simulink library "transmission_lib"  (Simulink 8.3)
settings: Solver=ode45  StartTime=0.0  StopTime=10.0  RelTol=1e-3
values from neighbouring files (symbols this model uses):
  dual_clutch = class_REVS_dual_clutch    [class_REVS_DCT_transmission.m]
  electric = class_REVS_electric(engine)    [electric_standard_car.m]
  gear = class_REVS_gearbox    [class_REVS_AMT_transmission.m]    (also in class_REVS_AT_transmission.m; class_REVS_CVT_transmission.m)
  torque_converter = class_REVS_torque_converter    [class_REVS_AT_transmission.m]    (also in class_REVS_CVT_transmission.m)
  transmission = class_REVS_AT_transmission    [transmission_6AT.m]    (also in transmission_8DCT.m = class_REVS_DCT_transmission; transmission_CVT.m = class_REVS_CVT_transmission)
undefined symbols (not defined in the file or in its folder): clutch, convert, gear_strategy, InitialSpeed_radps, LoadSource, SpeedSource, Value
libraries: general_lib x129, simulink x57, transmission_lib x50, audit_lib x11
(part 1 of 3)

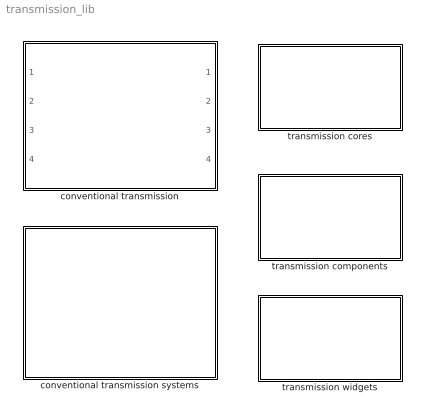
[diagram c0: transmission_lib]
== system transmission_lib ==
  conventional transmission : Subsystem  Variant=on
  conventional transmission systems : Subsystem
  transmission components : Subsystem
  transmission cores : Subsystem
  transmission widgets : Subsystem

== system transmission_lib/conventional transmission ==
  note: 1) Only subsystems can be added as variant choices at this level 2) Blocks cannot be connected at this level as connectivity is automatically determined at simulation, based on the active variant
  system_bus : Inport
  trq_in_Nm : Inport  Port=2
  iner_in_kgm2 : Inport  Port=3
  spd_out_radps : Inport  Port=4
  CVT transmission. system : transmission_lib/conventional transmission systems/CVT transmission system  VariantControl=transmission_type == enum_transmission_type.CVT
  automatic transmission system : transmission_lib/conventional transmission systems/automatic transmission system  VariantControl=transmission_type == enum_transmission_type.automatic
  dct transmission system : transmission_lib/conventional transmission systems/dct transmission system  VariantControl=transmission_type == enum_transmission_type.DCT
  bus_out : Outport
  trq_out_Nm : Outport  Port=2
  iner_out_kgm2 : Outport  Port=3
  spd_in_radps : Outport  Port=4

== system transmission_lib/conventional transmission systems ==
  CVT trans control : Subsystem  VariantControl=variants_trans_control_default
  CVT transmission system : Subsystem  VariantControl=transmission_type == enum_transmission_type.CVT
  automatic trans control : Subsystem  VariantControl=variants_trans_control_default
  automatic transmission system : Subsystem  VariantControl=transmission_type == enum_transmission_type.automatic
  dct trans control : Subsystem  VariantControl=variants_trans_control_manual
  dct transmission system : Subsystem  VariantControl=transmission_type == enum_transmission_type.DCT

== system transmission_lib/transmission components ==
  clutch : Subsystem
  dual clutch module : Subsystem
  gearbox : Subsystem
  simple gear : Subsystem
  torque converter : Subsystem

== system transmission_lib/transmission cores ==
  automatic core control : Subsystem  VariantControl=variants_trans_automatic
  automatic transmission core : Subsystem  VariantControl=variants_trans_automatic
  core control : Subsystem  Variant=on
  dct core control : Subsystem  VariantControl=variants_trans_dct
  dct transmission core : Subsystem  VariantControl=variants_trans_manual
  transmission cores : Subsystem  Variant=on

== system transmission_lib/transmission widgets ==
  auto neutral logic : Subsystem
  delayed lockup : Subsystem
  engage target speed calc : Subsystem
  gear select : Subsystem  Variant=on
  gear select variants : Subsystem
  load select : Subsystem
  lockup select : Subsystem  Variant=on
  lockup select variants : Subsystem
  low speed clutch engagement : Subsystem
  shift counter : Subsystem
  speed select : Subsystem
  thermal model : Subsystem  Variant=on
  thermal variants : Subsystem

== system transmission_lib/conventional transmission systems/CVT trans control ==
  system_bus : Inport
  Auto Neutral : Product  Inputs=**
  Bus Creator : BusCreator  Inputs=10
  Bus Selector : BusSelector  OutputSignals=driver.driver_acl_norm
  Bus Selector1 : BusSelector  OutputSignals=powertrain.trans.core.gearbox.gb_curr_gear
  Compare To Zero : simulink/Logic and Bit Operations/Compare To Zero  relop=>  OutDataTypeStr=boolean  ZeroCross=off
  Logical Operator1 : Logic  Operator=NOT  AllPortsSameDT=off  OutDataTypeStr=boolean
  auto neutral logic : transmission_lib/transmission widgets/auto neutral logic
  comp_iner_enable1 : Constant  Value=Inf
  driver acl to eng des acl : Gain
  gb curr gear to tans curr gear : Gain
  gear select : transmission_lib/transmission widgets/gear select
  line pressure control : Subsystem
  lockup select : transmission_lib/transmission widgets/lockup select
  to datalog : general_lib/to datalog  VarName=transmission__torque_converter_clutch_command_norm  WorkspaceName=datalog__transmission__torque_converter_clutch_command_norm  VerboseLevel=1  VerboseSignal=REVS.verbose
  to datalog1 : general_lib/to datalog  VarName=transmission__selected_gear_num  WorkspaceName=datalog__transmission__selected_gear_num  VerboseLevel=0  VerboseSignal=REVS.verbose
  to datalog2 : general_lib/to datalog  VarName=transmission__command_line_pressure_bar  WorkspaceName=datalog__transmission__command_line_pressure_bar  VerboseLevel=1  VerboseSignal=REVS.verbose
  to datalog5 : general_lib/to datalog  VarName=transmission__current_gear  WorkspaceName=datalog__transmission__current_gear  VerboseLevel=1  VerboseSignal=REVS.verbose
  trans des eng spd : Constant  Value=0
  trans des eng spd1 : Constant  Value=0
  upshift inertia compensation : Subsystem
  bus_out : Outport
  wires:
  auto neutral logic/1 -> Logical Operator1/1
  gear select/1 -> Auto Neutral/1
  Logical Operator1/1 -> Auto Neutral/2
  gb curr gear to tans curr gear/1 -> Bus Creator/9, to datalog5/1  "trans_curr_gear"
  line pressure control/1(cmd_line_press_bar) -> Bus Creator/8, to datalog2/1  "gb_line_press_bar"
  comp_iner_enable1/1 -> Bus Creator/7  "eng_des_load_limit_Nm"
  upshift inertia compensation/1(comp_iner_enable) -> Bus Creator/6  "eng_comp_iner_enable"
  Bus Selector1/1 -> lockup select/1, gb curr gear to tans curr gear/1  "<gb_curr_gear>"
  Bus Selector/1 -> driver acl to eng des acl/1  "<driver_acl_norm>"
  Auto Neutral/1 -> to datalog1/1, Compare To Zero/1, Bus Creator/1  "gear_num"
  system_bus/1 -> Bus Selector1/1, line pressure control/1(system_bus), upshift inertia compensation/1(system_bus), Bus Selector/1, lockup select/2, auto neutral logic/1, gear select/1
  Bus Creator/1 -> bus_out/1  "ctrl"
  lockup select/1 -> Bus Creator/3, to datalog/1  "tcc_lockup_cmd_bool"
  driver acl to eng des acl/1 -> Bus Creator/5  "eng_des_acl_norm"
  trans des eng spd/1 -> Bus Creator/4  "eng_des_spd_radps"
  Compare To Zero/1 -> Bus Creator/2  "driveline_engaged_bool"
  trans des eng spd1/1 -> Bus Creator/10  "trans_shift_in_prog"

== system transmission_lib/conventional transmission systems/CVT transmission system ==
  system_bus : Inport
  trq_in_Nm : Inport  Port=2
  iner_in_kgm2 : Inport  Port=3
  spd_out_radps : Inport  Port=4
  Bus Creator : BusCreator
  CVT trans control : transmission_lib/conventional transmission systems/CVT trans control  VariantControl=variants_trans_control_default
  automatic transmission core : transmission_lib/transmission cores/automatic transmission core  VariantControl=variants_trans_automatic
  result work : general_lib/result work  ResultSignalName=transmission_output_pos_work_kJ
  thermal model : transmission_lib/transmission widgets/thermal model
  to datalog : general_lib/to datalog  VarName=transmission.output_torque_Nm  WorkspaceName=datalog__transmission__output_torque_Nm  VerboseLevel=0  VerboseSignal=REVS.verbose
  to datalog1 : general_lib/to datalog  VarName=transmission.output_inertia_kgm2  WorkspaceName=datalog__transmission__output_inertia_kgm2  VerboseLevel=0  VerboseSignal=REVS.verbose
  to datalog2 : general_lib/to datalog  VarName=transmission.output_speed_radps  WorkspaceName=datalog__transmission__output_speed_radps  VerboseLevel=0  VerboseSignal=REVS.verbose
  torque converter : transmission_lib/transmission components/torque converter  base_name=torque_converter  torque_converter=transmission.torque_converter  pump_loss_Nm=transmission.pump_loss_Nm  pump_loss_base_name=torque_converter__pumploss  InitialSpeed_radps=0
  bus_out : Outport
  trq_out_Nm : Outport  Port=2
  iner_out_kgm2 : Outport  Port=3
  spd_in_radps : Outport  Port=4
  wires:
  spd_out_radps/1 -> to datalog2/1, automatic transmission core/4, result work/2
  torque converter/1 -> Bus Creator/3  "trq_conv"
  Bus Creator/1 -> torque converter/1, automatic transmission core/1, bus_out/1  "trans"
  system_bus/1 -> thermal model/1, CVT trans control/1
  CVT trans control/1 -> Bus Creator/1  "ctrl"
  automatic transmission core/1 -> Bus Creator/4  "core"
  automatic transmission core/2 -> to datalog/1, trq_out_Nm/1, result work/1
  automatic transmission core/3 -> result work/3, to datalog1/1, iner_out_kgm2/1
  trq_in_Nm/1 -> torque converter/2
  iner_in_kgm2/1 -> torque converter/3
  torque converter/2 -> automatic transmission core/2
  torque converter/3 -> automatic transmission core/3
  torque converter/4 -> spd_in_radps/1
  automatic transmission core/4 -> torque converter/4
  thermal model/1 -> Bus Creator/2  "therm"

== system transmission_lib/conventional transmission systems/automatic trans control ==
  system_bus : Inport
  Bus Creator : BusCreator  Inputs=10
  Bus Selector1 : BusSelector  OutputSignals=powertrain.trans.core.gearbox.gb_curr_gear
  Bus Selector2 : BusSelector  OutputSignals=driver.driver_acl_norm
  Compare To Zero : simulink/Logic and Bit Operations/Compare To Zero  relop=>  OutDataTypeStr=boolean  ZeroCross=off
  Divide : Product  Inputs=**
  Logical Operator1 : Logic  Operator=NOT  AllPortsSameDT=off  OutDataTypeStr=boolean
  Saturation : Saturate  UpperLimit=1  LowerLimit=-1
  Sum : Sum  Inputs=+-
  auto neutral logic : transmission_lib/transmission widgets/auto neutral logic
  comp_iner_enable1 : Constant  Value=Inf
  driver acl to eng des acl : Gain
  gb curr gear to tans curr gear : Gain
  gear select : transmission_lib/transmission widgets/gear select
  line pressure control : Subsystem
  lockup select : transmission_lib/transmission widgets/lockup select
  shift counter : transmission_lib/transmission widgets/shift counter
  to datalog : general_lib/to datalog  VarName=transmission__torque_converter_clutch_command_norm  WorkspaceName=datalog__transmission__torque_converter_clutch_command_norm  VerboseLevel=1  VerboseSignal=REVS.verbose
  to datalog1 : general_lib/to datalog  VarName=transmission__selected_gear_num  WorkspaceName=datalog__transmission__selected_gear_num  VerboseLevel=0  VerboseSignal=REVS.verbose
  to datalog2 : general_lib/to datalog  VarName=transmission__command_line_pressure_bar  WorkspaceName=datalog__transmission__command_line_pressure_bar  VerboseLevel=1  VerboseSignal=REVS.verbose
  to datalog5 : general_lib/to datalog  VarName=transmission__current_gear  WorkspaceName=datalog__transmission__current_gear  VerboseLevel=1  VerboseSignal=REVS.verbose
  trans des eng spd : Constant  Value=0
  upshift inertia compensation : Subsystem
  bus_out : Outport
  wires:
  Saturation/1 -> Bus Creator/9  "trans_shift_in_prog"
  Sum/1 -> Saturation/1
  Logical Operator1/1 -> Divide/2
  auto neutral logic/1 -> Logical Operator1/1
  gear select/1 -> Divide/1, to datalog1/1
  Compare To Zero/1 -> Bus Creator/2  "driveline_engaged_bool"
  trans des eng spd/1 -> Bus Creator/6  "eng_des_spd_radps"
  driver acl to eng des acl/1 -> Bus Creator/5  "eng_des_acl_norm"
  lockup select/1 -> to datalog/1, Bus Creator/3  "tcc_lockup_cmd_bool"
  Bus Creator/1 -> bus_out/1  "ctrl"
  system_bus/1 -> Bus Selector2/1, line pressure control/1(system_bus), Bus Selector1/1, upshift inertia compensation/1(system_bus), lockup select/2, auto neutral logic/1, gear select/1
  Divide/1 -> shift counter/1, Sum/1, Compare To Zero/1, Bus Creator/1  "gear_num"
  comp_iner_enable1/1 -> Bus Creator/7  "eng_des_load_limit_Nm"
  line pressure control/1(cmd_line_press_bar) -> Bus Creator/8, to datalog2/1  "gb_line_press_bar"
  gb curr gear to tans curr gear/1 -> Sum/2, Bus Creator/10, to datalog5/1  "trans_curr_gear"
  Bus Selector1/1 -> gb curr gear to tans curr gear/1, lockup select/1  "<gb_curr_gear>"
  Bus Selector2/1 -> driver acl to eng des acl/1  "<driver_acl_norm>"
  upshift inertia compensation/1(comp_iner_enable) -> Bus Creator/4  "eng_comp_iner_enable"

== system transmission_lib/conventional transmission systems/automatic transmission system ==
  system_bus : Inport
  trq_in_Nm : Inport  Port=2
  iner_in_kgm2 : Inport  Port=3
  spd_out_radps : Inport  Port=4
  Bus Creator : BusCreator
  automatic trans control : transmission_lib/conventional transmission systems/automatic trans control  VariantControl=variants_trans_control_default
  automatic transmission core : transmission_lib/transmission cores/automatic transmission core  VariantControl=variants_trans_automatic
  result work : general_lib/result work  ResultSignalName=transmission_output_pos_work_kJ
  thermal model : transmission_lib/transmission widgets/thermal model
  to datalog : general_lib/to datalog  VarName=transmission.output_torque_Nm  WorkspaceName=datalog__transmission__output_torque_Nm  VerboseLevel=0  VerboseSignal=REVS.verbose
  to datalog1 : general_lib/to datalog  VarName=transmission.output_inertia_kgm2  WorkspaceName=datalog__transmission__output_inertia_kgm2  VerboseLevel=0  VerboseSignal=REVS.verbose
  to datalog2 : general_lib/to datalog  VarName=transmission.output_speed_radps  WorkspaceName=datalog__transmission__output_speed_radps  VerboseLevel=0  VerboseSignal=REVS.verbose
  torque converter : transmission_lib/transmission components/torque converter  base_name=torque_converter  torque_converter=transmission.torque_converter  pump_loss_Nm=transmission.pump_loss_Nm  pump_loss_base_name=torque_converter__pumploss  InitialSpeed_radps=0
  bus_out : Outport
  trq_out_Nm : Outport  Port=2
  iner_out_kgm2 : Outport  Port=3
  spd_in_radps : Outport  Port=4
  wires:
  torque converter/1 -> Bus Creator/3  "trq_conv"
  Bus Creator/1 -> automatic transmission core/1, torque converter/1, bus_out/1  "trans"
  system_bus/1 -> thermal model/1, automatic trans control/1
  automatic trans control/1 -> Bus Creator/1  "ctrl"
  automatic transmission core/1 -> Bus Creator/4  "core"
  automatic transmission core/2 -> trq_out_Nm/1, result work/1, to datalog/1
  automatic transmission core/3 -> to datalog1/1, result work/3, iner_out_kgm2/1
  trq_in_Nm/1 -> torque converter/2
  iner_in_kgm2/1 -> torque converter/3
  torque converter/2 -> automatic transmission core/2
  torque converter/3 -> automatic transmission core/3
  spd_out_radps/1 -> automatic transmission core/4, result work/2, to datalog2/1  "trans_spd_out_radps"
  torque converter/4 -> spd_in_radps/1
  automatic transmission core/4 -> torque converter/4
  thermal model/1 -> Bus Creator/2  "therm"

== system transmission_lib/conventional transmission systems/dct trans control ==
  system_bus : Inport
  Bus Creator : BusCreator  Inputs=7
  Bus Selector : BusSelector  OutputSignals=powertrain.engine.eng_spd_radps,powertrain.trans.core.trans_spd_out_radps,driver.driver_acl_norm,driver.driver_brk_norm,powertrain.trans.ctrl.core_ctl.trans_shift_in_prog,powertrain.trans.core.dual_clutch.dct_capacity_Nm
  Bus Selector1 : BusSelector  OutputSignals=trans_curr_gear
  Compare To Zero : simulink/Logic and Bit Operations/Compare To Zero  relop=~=  OutDataTypeStr=boolean  ZeroCross=off
  Product2 : Product
  Saturation : Saturate  UpperLimit=1  LowerLimit=0
  dct cap to load limit : Gain
  dct core control : transmission_lib/transmission cores/dct core control  VariantControl=variants_trans_dct
  driver acl to eng des acl : Gain
  gear ratio : LookupNDDirect  NumberOfTableDimensions=1  Table=transmission.gear.ratio
  gear select : transmission_lib/transmission widgets/gear select
  low speed clutch engagement1 : transmission_lib/transmission widgets/low speed clutch engagement  clutch=transmission.control
  shift counter : transmission_lib/transmission widgets/shift counter
  trans des eng spd : Constant  Value=0
  bus_out : Outport
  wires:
  Bus Selector/6 -> dct cap to load limit/1  "<dct_capacity_Nm>"
  Bus Selector/5 -> Saturation/1  "<trans_shift_in_prog>"
  dct cap to load limit/1 -> Bus Creator/7  "eng_des_load_limit_Nm"
  gear ratio/1 -> Product2/1
  Bus Selector/2 -> Product2/2  "<trans_spd_out_radps>"
  Bus Selector/3 -> low speed clutch engagement1/3, driver acl to eng des acl/1  "<driver_acl_norm>"
  system_bus/1 -> Bus Selector/1, dct core control/1, gear select/1
  Bus Creator/1 -> bus_out/1  "ctrl"
  trans des eng spd/1 -> Bus Creator/5  "eng_des_spd_radps"
  driver acl to eng des acl/1 -> Bus Creator/4  "eng_des_acl_norm"
  Bus Selector/1 -> low speed clutch engagement1/1  "<eng_spd_radps>"
  Product2/1 -> low speed clutch engagement1/2
  Bus Selector/4 -> low speed clutch engagement1/4  "<driver_brk_norm>"
  Saturation/1 -> Bus Creator/6  "eng_comp_iner_enable"
  Compare To Zero/1 -> low speed clutch engagement1/6
  dct core control/1 -> Bus Selector1/1, Bus Creator/3  "core_ctl"
  low speed clutch engagement1/1 -> Bus Creator/1  "clutch_cmd_norm"
  gear select/1 -> gear ratio/1, Bus Creator/2, Compare To Zero/1, low speed clutch engagement1/5  "gear_num"
  Bus Selector1/1 -> shift counter/1  "<trans_curr_gear>"

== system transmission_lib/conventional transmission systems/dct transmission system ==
  system_bus : Inport
  trq_in_Nm : Inport  Port=2
  iner_in_kgm2 : Inport  Port=3
  spd_out_radps : Inport  Port=4
  Bus Creator : BusCreator  Inputs=3
  dct trans control : transmission_lib/conventional transmission systems/dct trans control  VariantControl=variants_trans_control_manual
  dct transmission core : transmission_lib/transmission cores/dct transmission core  VariantControl=variants_trans_manual
  result work : general_lib/result work  ResultSignalName=transmission_output_pos_work_kJ
  thermal model : transmission_lib/transmission widgets/thermal model
  to datalog : general_lib/to datalog  VarName=transmission.output_torque_Nm  WorkspaceName=datalog__transmission__output_torque_Nm  VerboseLevel=0  VerboseSignal=REVS.verbose
  to datalog1 : general_lib/to datalog  VarName=transmission.output_inertia_kgm2  WorkspaceName=datalog__transmission__output_inertia_kgm2  VerboseLevel=0  VerboseSignal=REVS.verbose
  to datalog2 : general_lib/to datalog  VarName=transmission.output_speed_radps  WorkspaceName=datalog__transmission__output_speed_radps  VerboseLevel=0  VerboseSignal=REVS.verbose
  bus_out : Outport
  trq_out_Nm : Outport  Port=2
  iner_out_kgm2 : Outport  Port=3
  spd_in_radps : Outport  Port=4
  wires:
  iner_in_kgm2/1 -> dct transmission core/3
  spd_out_radps/1 -> to datalog2/1, result work/2, dct transmission core/4
  trq_in_Nm/1 -> dct transmission core/2
  dct transmission core/4 -> spd_in_radps/1
  dct transmission core/3 -> result work/3, to datalog1/1, iner_out_kgm2/1
  dct transmission core/2 -> trq_out_Nm/1, result work/1, to datalog/1
  system_bus/1 -> dct trans control/1, thermal model/1
  dct trans control/1 -> Bus Creator/1  "ctrl"
  dct transmission core/1 -> Bus Creator/3  "core"
  thermal model/1 -> Bus Creator/2  "therm"
  Bus Creator/1 -> dct transmission core/1, bus_out/1  "trans"

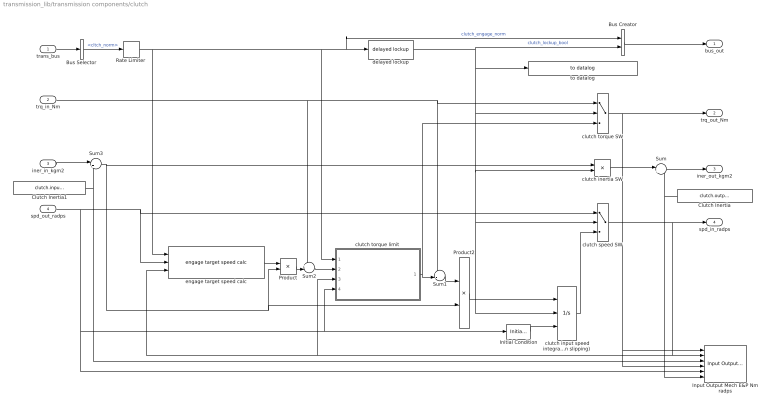
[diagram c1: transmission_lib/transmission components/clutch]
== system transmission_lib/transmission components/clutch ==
  trans_bus : Inport
  trq_in_Nm : Inport  Port=2
  iner_in_kgm2 : Inport  Port=3
  spd_out_radps : Inport  Port=4
  " clutch input speed integrator  (integrate when slipping)" : Integrator  ExternalReset=falling  InitialConditionSource=external  LimitOutput=on  UpperSaturationLimit=Inf  LowerSaturationLimit=0
  Bus Creator : BusCreator  Inputs=2
  Bus Selector : BusSelector  OutputSignals=cltch_norm
  Clutch Inertia : Constant  Value=clutch.output_inertia_kgm2
  Clutch Inertia1 : Constant  Value=clutch.input_inertia_kgm2
  Initial Condition : general_lib/Initial Condition  InitialValue=InitialSpeed_radps
  Input Output Mech E&P Nm radps : audit_lib/Input Output Mech E&P Nm radps  base_name=clutch  VerboseSignal=REVS.verbose
  Product : Product
  Product2 : Product  Inputs=*/
  Rate Limiter : RateLimiter  RisingSlewLimit=1/clutch.engage_duration_secs  FallingSlewLimit=-inf  SampleTimeMode=inherited
  Sum : Sum  Inputs=|++
  Sum1 : Sum  Inputs=+-|
  Sum2 : Sum  Inputs=+-|
  Sum3 : Sum  Inputs=|++
  clutch inertia SW : Product
  clutch speed SW : Switch  Threshold=1
  clutch torque SW : Switch  Threshold=1
  clutch torque limit : Subsystem
  delayed lockup : transmission_lib/transmission widgets/delayed lockup
  engage target speed calc : transmission_lib/transmission widgets/engage target speed calc
  to datalog : general_lib/to datalog  VarName=transmission__clutch_lockup_bool  WorkspaceName=datalog__transmission__clutch_lockup_bool  VerboseLevel=1  VerboseSignal=REVS.verbose
  bus_out : Outport
  trq_out_Nm : Outport  Port=2
  iner_out_kgm2 : Outport  Port=3
  spd_in_radps : Outport  Port=4
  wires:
  Rate Limiter/1 -> clutch torque limit/1(engage), Bus Creator/1, delayed lockup/1, engage target speed calc/1  "clutch_engage_norm"
  delayed lockup/1 -> clutch inertia SW/2, " clutch input speed integrator  (integrate when slipping)"/2, clutch speed SW/2, clutch torque SW/2, to datalog/1, Bus Creator/2  "clutch_lockup_bool"
  Product2/1 -> " clutch input speed integrator  (integrate when slipping)"/1
  Product/1 -> Sum2/2
  spd_out_radps/1 -> clutch speed SW/1, engage target speed calc/2, Initial Condition/1, clutch torque limit/4(output_speed_radps), Input Output Mech E&P Nm radps/5
  " clutch input speed integrator  (integrate when slipping)"/1 -> clutch speed SW/3
  trq_in_Nm/1 -> Sum1/1, clutch torque SW/1, Sum2/1
  Sum3/1 -> clutch inertia SW/1, Product/2, Product2/2
  engage target speed calc/1 -> Product/1
  Sum1/1 -> Product2/1
  clutch speed SW/1 -> clutch torque limit/3(input_speed_radps), engage target speed calc/3, Input Output Mech E&P Nm radps/2, spd_in_radps/1
  clutch torque SW/1 -> trq_out_Nm/1, Input Output Mech E&P Nm radps/4, Input Output Mech E&P Nm radps/1
  trans_bus/1 -> Bus Selector/1
  clutch inertia SW/1 -> Sum/1
  Sum/1 -> iner_out_kgm2/1
  Clutch Inertia/1 -> Input Output Mech E&P Nm radps/6, Sum/2
  iner_in_kgm2/1 -> Sum3/1
  Clutch Inertia1/1 -> Input Output Mech E&P Nm radps/3, Sum3/2
  Initial Condition/1 -> " clutch input speed integrator  (integrate when slipping)"/3
  clutch torque limit/1(lim_transmit_torque_Nm) -> Sum1/2, clutch torque SW/3
  Sum2/1 -> clutch torque limit/2("req_transmit_torque_Nm ")
  Bus Creator/1 -> bus_out/1
  Bus Selector/1 -> Rate Limiter/1  "<cltch_norm>"

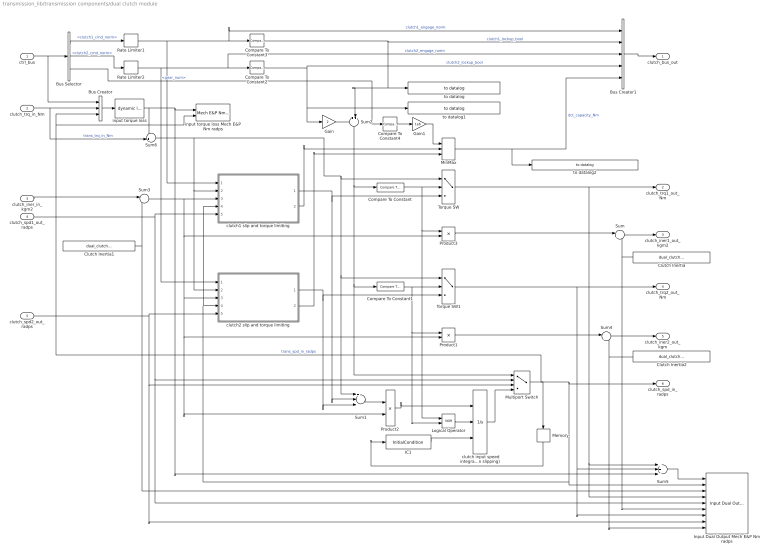
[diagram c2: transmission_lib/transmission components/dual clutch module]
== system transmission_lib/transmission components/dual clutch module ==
  ctrl_bus : Inport
  clutch_trq_in_Nm : Inport  Port=2
  clutch_iner_in_kgm2 : Inport  Port=3
  clutch_spd1_out_radps : Inport  Port=4
  clutch_spd2_out_radps : Inport  Port=5
  " clutch input speed integrator  (integrate when slipping)" : Integrator  ExternalReset=rising  InitialConditionSource=external  LimitOutput=on  UpperSaturationLimit=Inf  LowerSaturationLimit=0
  Bus Creator : BusCreator  Inputs=3
  Bus Creator1 : BusCreator  Inputs=5
  Bus Selector : BusSelector  OutputSignals=ctrl.core_ctl.clutch1_cmd_norm,ctrl.core_ctl.clutch2_cmd_norm,ctrl.gear_num
  Clutch Inertia : Constant  Value=dual_clutch.output1_inertia_kgm2
  Clutch Inertia1 : Constant  Value=dual_clutch.input_inertia_kgm2
  Clutch Inertia2 : Constant  Value=dual_clutch.output2_inertia_kgm2
  Compare To Constant{,2..4} (4 alike) : simulink/Logic and Bit Operations/Compare To Constant  relop===  const=1  OutDataTypeStr=boolean
  Compare To Constant1 : simulink/Logic and Bit Operations/Compare To Constant  relop===  const=2  OutDataTypeStr=boolean
  Gain : Gain  Gain=2
  Gain1 : Gain  Gain=1e6
  IC1 : InitialCondition  Value=InitialSpeed_radps
  Input Dual Output Mech E&P Nm radps : audit_lib/Input Dual Output Mech E&P Nm radps  base_name=dual_clutch  VerboseSignal=REVS.verbose
  Logical Operator : Logic  Operator=NOR  AllPortsSameDT=off  OutDataTypeStr=boolean
  Memory : Memory  X0=InitialSpeed_radps
  MinMax : MinMax  Function=max  Inputs=3
  Multiport Switch : MultiPortSwitch  Inputs=2  DataPortForDefault=Additional data port  DiagnosticForDefault=None
  Product1 : Product
  Product2 : Product  Inputs=*/
  Product3 : Product
  Rate Limiter1 : RateLimiter  RisingSlewLimit=1/dual_clutch.engage_duration_secs  FallingSlewLimit=-inf  SampleTimeMode=inherited
  Rate Limiter2 : RateLimiter  RisingSlewLimit=1/dual_clutch.engage_duration_secs  FallingSlewLimit=-inf  SampleTimeMode=inherited
  Sum : Sum  Inputs=|++
  Sum1 : Sum  Inputs=+--
  Sum2 : Sum  Inputs=++|
  Sum3 : Sum  Inputs=|++
  Sum4 : Sum  Inputs=|++
  Sum5 : Sum  Inputs=+++
  Sum6 : Sum  Inputs=-+|
  Torque SW : Switch  Threshold=1
  Torque SW1 : Switch  Threshold=1
  clutch1 slip and torque limiting : Subsystem
  clutch2 slip and torque limiting : Subsystem
  input torque loss : general_lib/dynamic lookup  LookupStructure=dual_clutch.input_torque_loss_Nm  InterpMethod=Linear  ExtrapMethod=Clip  DiagnosticForOutOfRangeInput=Warning  IndexSearchMethod=Linear search  BeginIndexSearchUsingPreviousIndexResult=on  SupportTunableTableSize=off  LookupStructureEval=|
      | LookupStructure =
      | 
      |      []
  input torque loss Mech E&P Nm radps : audit_lib/Mech E&P Nm radps0  base_name=dual_clutch.input_torque_loss  VerboseSignal=REVS.verbose
  to datalog : general_lib/to datalog  VarName=transmission__clutch1_lockup_bool  WorkspaceName=datalog__transmission__clutch1_lockup_bool  VerboseLevel=2  VerboseSignal=REVS.verbose
  to datalog1 : general_lib/to datalog  VarName=transmission__clutch2_lockup_bool  WorkspaceName=datalog__transmission__clutch2_lockup_bool  VerboseLevel=2  VerboseSignal=REVS.verbose
  to datalog2 : general_lib/to datalog  VarName=transmission__dual_clutch_capacity_Nm  WorkspaceName=datalog__transmission__dual_clutch_capacity_Nm  VerboseLevel=2  VerboseSignal=REVS.verbose
  clutch_bus_out : Outport
  clutch_trq1_out_Nm : Outport  Port=2
  clutch_iner1_out_kgm2 : Outport  Port=3
  clutch_trq2_out_Nm : Outport  Port=4
  clutch_iner2_out_kgm : Outport  Port=5
  clutch_spd_in_radps : Outport  Port=6
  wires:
  Gain1/1 -> MinMax/1
  Compare To Constant4/1 -> Gain1/1
  Bus Selector/3 -> Compare To Constant4/1  "<gear_num>"
  clutch1 slip and torque limiting/2(torque_limit_Nm) -> MinMax/2
  clutch2 slip and torque limiting/2(torque_limit_Nm) -> MinMax/3
  MinMax/1 -> to datalog2/1, Bus Creator1/5  "dct_capacity_Nm"
  Sum5/1 -> Input Dual Output Mech E&P Nm radps/1
  Multiport Switch/1 -> Memory/1, input torque loss Mech E&P Nm radps/2, Bus Creator/3, clutch1 slip and torque limiting/4(input_speed_radps), clutch2 slip and torque limiting/4(input_speed_radps), Input Dual Output Mech E&P Nm radps/2, clutch_spd_in_radps/1  "trans_spd_in_radps"
  clutch_trq_in_Nm/1 -> Sum6/2, Bus Creator/2  "trans_trq_in_Nm"
  input torque loss/1 -> input torque loss Mech E&P Nm radps/1, Sum5/3, Sum6/1
  Bus Creator/1 -> input torque loss/1
  Memory/1 -> IC1/1
  Logical Operator/1 -> " clutch input speed integrator  (integrate when slipping)"/2
  IC1/1 -> " clutch input speed integrator  (integrate when slipping)"/3
  Clutch Inertia1/1 -> Sum3/2, Input Dual Output Mech E&P Nm radps/3
  clutch_iner_in_kgm2/1 -> Sum3/1
  Clutch Inertia/1 -> Sum/2, Input Dual Output Mech E&P Nm radps/6
  Sum/1 -> clutch_iner1_out_kgm2/1
  Product3/1 -> Sum/1
  ctrl_bus/1 -> Bus Selector/1, Bus Creator/1
  Torque SW/1 -> Sum5/1, Input Dual Output Mech E&P Nm radps/4, clutch_trq1_out_Nm/1
  Sum1/1 -> Product2/1
  Sum3/1 -> Product3/2, clutch2 slip and torque limiting/3(inertia_kgm2), Product1/2, Product2/2, clutch1 slip and torque limiting/3(inertia_kgm2)
  " clutch input speed integrator  (integrate when slipping)"/1 -> Multiport Switch/4
  clutch_spd1_out_radps/1 -> Multiport Switch/2, Input Dual Output Mech E&P Nm radps/5, clutch1 slip and torque limiting/5(output_speed_radps)
  Product2/1 -> " clutch input speed integrator  (integrate when slipping)"/1
  Compare To Constant3/1 -> Bus Creator1/2, Sum2/2, to datalog/1  "clutch1_lockup_bool"
  Rate Limiter1/1 -> clutch1 slip and torque limiting/1(engage), Bus Creator1/1, Compare To Constant3/1  "clutch1_engage_norm"
  Torque SW1/1 -> Input Dual Output Mech E&P Nm radps/7, Sum5/2, clutch_trq2_out_Nm/1
  clutch1 slip and torque limiting/1(transmit_torque_Nm) -> Sum1/2, Torque SW/3
  clutch_spd2_out_radps/1 -> Multiport Switch/3, Input Dual Output Mech E&P Nm radps/8, clutch2 slip and torque limiting/5(output_speed_radps)
  Sum4/1 -> clutch_iner2_out_kgm/1
  Clutch Inertia2/1 -> Input Dual Output Mech E&P Nm radps/9, Sum4/2
  Product1/1 -> Sum4/1
  Compare To Constant2/1 -> Gain/1, to datalog1/1, Bus Creator1/4  "clutch2_lockup_bool"
  clutch2 slip and torque limiting/1(transmit_torque_Nm) -> Sum1/3, Torque SW1/3
  Gain/1 -> Sum2/1
  Sum2/1 -> Multiport Switch/1, Compare To Constant1/1, Compare To Constant/1
  Compare To Constant/1 -> Logical Operator/1, Product3/1, Torque SW/2
  Compare To Constant1/1 -> Torque SW1/2, Logical Operator/2, Product1/1
  Sum6/1 -> clutch1 slip and torque limiting/2(input_torque_Nm), clutch2 slip and torque limiting/2(input_torque_Nm), Torque SW1/1, Sum1/1, Torque SW/1
  Bus Selector/1 -> Rate Limiter1/1  "<clutch1_cmd_norm>"
  Bus Selector/2 -> Rate Limiter2/1  "<clutch2_cmd_norm>"
  Rate Limiter2/1 -> clutch2 slip and torque limiting/1(engage), Bus Creator1/3, Compare To Constant2/1  "clutch2_engage_norm"
  Bus Creator1/1 -> clutch_bus_out/1

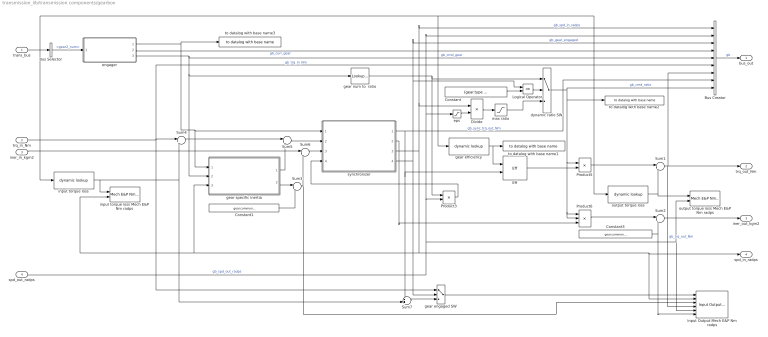
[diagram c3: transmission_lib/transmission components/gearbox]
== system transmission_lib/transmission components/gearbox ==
  trans_bus : Inport
  trq_in_Nm : Inport  Port=2
  iner_in_kgm2 : Inport  Port=3
  spd_out_radps : Inport  Port=4
  Bus Creator : BusCreator  Inputs=9
  Bus Selector : BusSelector  OutputSignals=gear2_num
  Constant : Constant  Value=(gear.type == enum_transmission_type.AMT) || (gear.type == enum_transmission_type.manual) || (gear.type == enum_transmission_type.DCT)
  Constant1 : Constant  Value=gear.common_input_inertia_kgm2
  Constant3 : Constant  Value=gear.common_output_inertia_kgm2
  Divide : Product  Inputs=*/
  Eff : general_lib/Eff
  Input Output Mech E&P Nm radps : audit_lib/Input Output Mech E&P Nm radps  base_name=gearbox2  VerboseSignal=REVS.verbose
  Logical Operator : Logic  Operator=OR  AllPortsSameDT=off  OutDataTypeStr=boolean
  Product3 : Product
  Product5 : Product
  Product6 : Product  Inputs=3
  Sum1 : Sum  Inputs=|+-
  Sum2 : Sum  Inputs=|++
  Sum3 : Sum  Inputs=|++
  Sum4 : Sum  Inputs=|+-
  Sum5 : Sum  Inputs=|+-
  Sum6 : Sum  Inputs=|++
  Sum7 : Sum  Inputs=++|
  dynamic ratio SW : Switch  Threshold=1
  engager : Subsystem
  eps : Saturate  UpperLimit=Inf  LowerLimit=1
  gear efficiency : general_lib/dynamic lookup  LookupStructure=gear.efficiency_norm  InterpMethod=Linear  ExtrapMethod=Linear  DiagnosticForOutOfRangeInput=Warning  IndexSearchMethod=Linear search  BeginIndexSearchUsingPreviousIndexResult=on  SupportTunableTableSize=off  LookupStructureEval=|
      | LookupStructure =
      | 
      |      []
  gear engaged SW : Switch  Threshold=1
  gear num to  ratio : Lookup_n-D  NumberOfTableDimensions=1  BreakpointsForDimension1=gear.number  IndexSearchMethod=Linear search  BeginIndexSearchUsingPreviousIndexResult=on  Table=gear.ratio  ExtrapMethod=Clip  DiagnosticForOutOfRangeInput=Error  InternalRulePriority=Speed  RndMeth=Simplest
  gear specific inertia : Subsystem
  input torque loss : general_lib/dynamic lookup  LookupStructure=gear.input_torque_loss_Nm  InterpMethod=Linear  ExtrapMethod=Linear  DiagnosticForOutOfRangeInput=None  IndexSearchMethod=Linear search  BeginIndexSearchUsingPreviousIndexResult=on  SupportTunableTableSize=off  LookupStructureEval=|
      | LookupStructure =
      | 
      |      []
  input torque loss Mech E&P Nm radps : audit_lib/Mech E&P Nm radps0  base_name=gearbox2__input_torque_loss  VerboseSignal=REVS.verbose
  max ratio : Saturate  UpperLimit=max(gear.ratio)  LowerLimit=0
  output torque loss : general_lib/dynamic lookup  LookupStructure=gear.output_torque_loss_Nm  InterpMethod=Linear  ExtrapMethod=Linear  DiagnosticForOutOfRangeInput=Warning  IndexSearchMethod=Linear search  BeginIndexSearchUsingPreviousIndexResult=on  SupportTunableTableSize=off  LookupStructureEval=|
      | LookupStructure =
      | 
      |      []
  output torque loss Mech E&P Nm radps : audit_lib/Mech E&P Nm radps0  base_name=gearbox2__output_torque_loss  VerboseSignal=REVS.verbose
  synchronizer : Subsystem
  to datalog with base name1 : general_lib/to datalog with base name  varName=gear_efficiency_norm  baseName=GearboxBaseName  VerboseLevel=1  VerboseSignal=REVS.verbose
  to datalog with base name2 : general_lib/to datalog with base name  varName=actual_ratio  baseName=GearboxBaseName  VerboseLevel=1  VerboseSignal=REVS.verbose
  to datalog with base name3 : general_lib/to datalog with base name  varName=engage_norm  baseName=GearboxBaseName  VerboseLevel=1  VerboseSignal=REVS.verbose
  bus_out : Outport
  trq_out_Nm : Outport  Port=2
  iner_out_kgm2 : Outport  Port=3
  spd_in_radps : Outport  Port=4
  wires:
  engager/2(curr_gear_num) -> Bus Creator/4  "gb_curr_gear"
  gear num to  ratio/1 -> Product3/1, dynamic ratio SW/1
  gear specific inertia/2(iner_out_kgm2) -> Sum3/1
  Sum7/1 -> gear engaged SW/3
  synchronizer/4(sync_lockup) -> Logical Operator/1, Bus Creator/3, gear engaged SW/2  "gb_gear_engaged"
  Sum3/1 -> Sum6/2, Input Output Mech E&P Nm radps/3
  gear specific inertia/1(iner_trq_out_Nm) -> Sum5/2
  Sum5/1 -> synchronizer/2(sync_trq_in_Nm)
  trq_in_Nm/1 -> gear engaged SW/1, Bus Creator/6, Sum4/1  "gb_trq_in_Nm"
  Constant1/1 -> Sum3/2
  Sum2/1 -> iner_out_kgm2/1
  engager/1(engage) -> to datalog with base name3/1, synchronizer/1(engage), gear specific inertia/1(engage)
  synchronizer/2(sync_iner_out_kgm2) -> Product6/3
  synchronizer/1(sync_trq_out_Nm) -> Bus Creator/8, Eff/2, Sum7/1  "gb_sync_trq_out_Nm"
  Eff/1 -> Product5/2
  gear efficiency/1 -> Eff/1, to datalog with base name1/1
  Bus Creator/1 -> bus_out/1  "gb"
  synchronizer/3(sync_spd_in_radps) -> Input Output Mech E&P Nm radps/2, spd_in_radps/1, input torque loss Mech E&P Nm radps/2, gear specific inertia/3(iner_spd_out_radps), Divide/1, Bus Creator/1  "gb_spd_in_radps"
  Sum1/1 -> Input Output Mech E&P Nm radps/4, trq_out_Nm/1, Bus Creator/7  "gb_trq_out_Nm"
  iner_in_kgm2/1 -> Sum6/1
  Product6/1 -> Sum2/1
  Constant3/1 -> Sum2/2, Input Output Mech E&P Nm radps/6
  Sum4/1 -> Sum5/1
  Sum6/1 -> synchronizer/3(sync_iner_in_kgm2)
  engager/3(cmd_gear_num) -> gear num to  ratio/1, gear specific inertia/2(cmd_gear_num), Bus Creator/5  "gb_cmd_gear"
  Bus Selector/1 -> engager/1(tgt_gear_num)  "<gear2_num>"
  input torque loss/1 -> Sum4/2, Sum7/2, input torque loss Mech E&P Nm radps/1
  Product3/1 -> synchronizer/4(sync_spd_out_radps)
  gear engaged SW/1 -> Input Output Mech E&P Nm radps/1
  eps/1 -> Divide/2
  dynamic ratio SW/1 -> Bus Creator/9, to datalog with base name2/1, Product6/2, Product6/1, Product5/1  "gb_cmd_ratio"
  Logical Operator/1 -> dynamic ratio SW/2
  Constant/1 -> Logical Operator/2
  trans_bus/1 -> Bus Selector/1, input torque loss/1, gear efficiency/1, output torque loss/1
  spd_out_radps/1 -> Product3/2, eps/1, Bus Creator/2, Input Output Mech E&P Nm radps/5, output torque loss Mech E&P Nm radps/2  "gb_spd_out_radps"
  output torque loss/1 -> Sum1/2, output torque loss Mech E&P Nm radps/1
  Product5/1 -> Sum1/1
  max ratio/1 -> dynamic ratio SW/3
  Divide/1 -> max ratio/1

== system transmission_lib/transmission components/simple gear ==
  trq_in_Nm : Inport
  iner_in_kgm2 : Inport  Port=2
  spd_out_radps : Inport  Port=3
  Constant1 : Constant  Value=gear.input_inertia_kgm2
  Constant2 : Constant  Value=gear.ratio
  Constant3 : Constant  Value=gear.output_inertia_kgm2
  Constant4 : Constant  Value=gear.efficiency_norm
  Eff : general_lib/Eff
  Input Output Mech E&P Nm radps : audit_lib/Input Output Mech E&P Nm radps  base_name=gearbox  VerboseSignal=REVS.verbose
  Product3 : Product
  Product5 : Product
  Product6 : Product  Inputs=3
  Sum2 : Sum  Inputs=|++
  Sum6 : Sum  Inputs=|++
  trq_out_Nm : Outport
  iner_out_kgm2 : Outport  Port=2
  spd_in_radps : Outport  Port=3
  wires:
  Constant1/1 -> Input Output Mech E&P Nm radps/3, Sum6/2
  Sum2/1 -> iner_out_kgm2/1
  Eff/1 -> Product5/2
  Constant4/1 -> Eff/1
  spd_out_radps/1 -> Product3/2, Input Output Mech E&P Nm radps/5
  Product5/1 -> trq_out_Nm/1, Input Output Mech E&P Nm radps/4
  iner_in_kgm2/1 -> Sum6/1
  Product6/1 -> Sum2/1
  Constant3/1 -> Input Output Mech E&P Nm radps/6, Sum2/2
  Sum6/1 -> Product6/3
  trq_in_Nm/1 -> Input Output Mech E&P Nm radps/1, Eff/2
  Constant2/1 -> Product6/2, Product6/1, Product5/1, Product3/1
  Product3/1 -> Input Output Mech E&P Nm radps/2, spd_in_radps/1

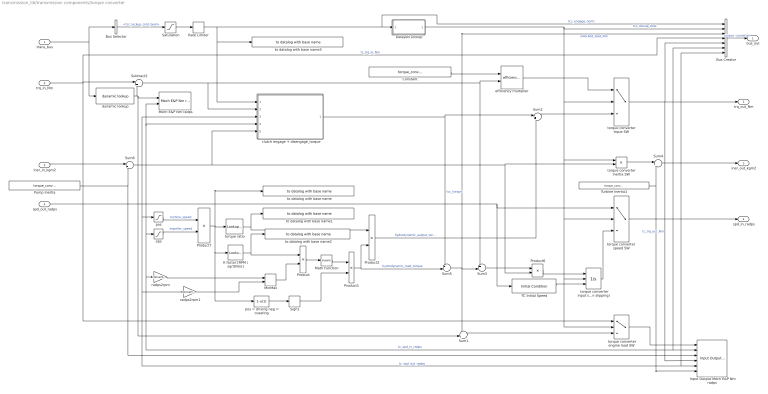
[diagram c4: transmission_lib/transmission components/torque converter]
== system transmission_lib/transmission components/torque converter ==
  trans_bus : Inport
  trq_in_Nm : Inport  Port=2
  iner_in_kgm2 : Inport  Port=3
  spd_out_radps : Inport  Port=4
  " torque converter engine load SW" : Switch  Threshold=0.5
  " torque converter input speed integrator  (integrate when slipping)" : Integrator  ExternalReset=falling  InitialConditionSource=external  LimitOutput=on  UpperSaturationLimit=Inf  LowerSaturationLimit=0
  Bus Selector : BusSelector  OutputSignals=ctrl.tcc_lockup_cmd_bool
  Bus Creator : BusCreator  Inputs=7
  Constant : Constant  Value=torque_converter.lockup_efficiency_norm
  Delayed Lockup : Subsystem
  Input Output Mech E&P Nm radps : audit_lib/Input Output Mech E&P Nm radps  base_name=torque_converter  VerboseSignal=REVS.verbose
  K factor [RPM / sqrt(Nm)] : Lookup_n-D  NumberOfTableDimensions=1  BreakpointsForDimension1=torque_converter.all_speed_ratios  IndexSearchMethod=Linear search  BeginIndexSearchUsingPreviousIndexResult=on  Table=torque_converter.all_k_factors_rpmpsqrtNm  ExtrapMethod=Clip  UseLastTableValue=on  InternalRulePriority=Speed  RndMeth=Simplest
  Math Function : Math  Operator=square
  Mech E&P Nm radps : audit_lib/Mech E&P Nm radps0  base_name=torque_converter__pumploss  VerboseSignal=REVS.verbose
  MinMax : MinMax  Function=max  Inputs=2  ZeroCross=off
  Product : Product  Inputs=/*
  Product1 : Product
  Product2 : Product
  Product6 : Product  Inputs=*/
  Product7 : Product  Inputs=*/
  Pump Inertia : Constant  Value=torque_converter.pump_inertia_kgm2
  Rate Limiter : RateLimiter  RisingSlewLimit=1/torque_converter.lockup_duration_secs  FallingSlewLimit=-1/torque_converter.unlock_duration_secs  InitialCondition=1
  Saturation : Saturate  UpperLimit=1  LowerLimit=0
  Sign1 : Signum  ZeroCross=off
  Subtract2 : Sum  Inputs=|+-
  Sum1 : Sum  Inputs=++|
  Sum2 : Sum  Inputs=|++
  Sum3 : Sum  Inputs=+-|
  Sum4 : Sum  Inputs=|++
  Sum5 : Sum  Inputs=++|
  Sum6 : Sum  Inputs=|++
  TC Initial Speed : general_lib/Initial Condition  InitialValue=InitialSpeed_radps
  Turbine Inertia1 : Constant  Value=torque_converter.turbine_inertia_kgm2
  clutch engage + disengage_torque : Subsystem
  dynamic lookup : general_lib/dynamic lookup  LookupStructure=pump_loss_Nm  InterpMethod=Linear  ExtrapMethod=Clip  DiagnosticForOutOfRangeInput=Warning  IndexSearchMethod=Linear search  BeginIndexSearchUsingPreviousIndexResult=on  SupportTunableTableSize=off  LookupStructureEval=|
      | LookupStructure =
      | 
      |      []
  efficiency multiplier : general_lib/efficiency multiplier  MultiplyPosInputs=true
  eps : Saturate  UpperLimit=inf  LowerLimit=eps
  pos : Saturate  UpperLimit=inf  LowerLimit=0
  pos = driving neg = coasting : Fcn  Expr=1-u(1)
  radps2rpm : Gain  Gain=convert.radps2rpm
  radps2rpm1 : Gain  Gain=convert.radps2rpm
  to datalog with base name : general_lib/to datalog with base name  varName=speed_ratio  baseName=base_name  VerboseLevel=2  VerboseSignal=REVS.verbose
  to datalog with base name1 : general_lib/to datalog with base name  varName=torque_ratio  baseName=base_name  VerboseLevel=2  VerboseSignal=REVS.verbose
  to datalog with base name2 : general_lib/to datalog with base name  varName=k_factor_rpmpsqrtNm  baseName=base_name  VerboseLevel=2  VerboseSignal=REVS.verbose
  to datalog with base name3 : general_lib/to datalog with base name  varName=tcc_engage_norm  baseName=base_name  VerboseLevel=2  VerboseSignal=REVS.verbose
  torque converter inertia SW : Product
  torque converter trque SW : Switch  Threshold=0.5
  torque converter  speed SW : Switch  Threshold=0.5
  torque ratio : Lookup_n-D  NumberOfTableDimensions=1  BreakpointsForDimension1=torque_converter.all_speed_ratios  IndexSearchMethod=Linear search  BeginIndexSearchUsingPreviousIndexResult=on  Table=torque_converter.all_torque_ratios  ExtrapMethod=Clip  UseLastTableValue=on  InternalRulePriority=Speed  RndMeth=Simplest
  bus_out : Outport
  trq_out_Nm : Outport  Port=2
  iner_out_kgm2 : Outport  Port=3
  spd_in_radps : Outport  Port=4
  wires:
  Saturation/1 -> Rate Limiter/1
  MinMax/1 -> Product/2
  dynamic lookup/1 -> Subtract2/2, Sum1/2, Mech E&P Nm radps/1
  Turbine Inertia1/1 -> Input Output Mech E&P Nm radps/6, Sum4/2
  Pump Inertia/1 -> Input Output Mech E&P Nm radps/3, Sum6/2
  torque ratio/1 -> to datalog with base name1/1, Product2/1
  Sum4/1 -> iner_out_kgm2/1
  Sum3/1 -> Product6/1
  torque converter inertia SW/1 -> Sum4/1
  torque converter trque SW/1 -> trq_out_Nm/1, Input Output Mech E&P Nm radps/4, Bus Creator/5  "tc_trq_out_Nm"
  " torque converter input speed integrator  (integrate when slipping)"/1 -> torque converter  speed SW/3
  Sign1/1 -> Product1/2
  Product1/1 -> Sum5/2, Product2/2  "hydrodynamic_load_torque"
  radps2rpm1/1 -> MinMax/2
  radps2rpm/1 -> MinMax/1
  pos = driving neg = coasting/1 -> Sign1/1
  Math Function/1 -> Product1/1
  Product/1 -> Math Function/1
  Subtract2/1 -> clutch engage + disengage_torque/2(trq_in_Nm), efficiency multiplier/2, Sum3/1
  torque converter  speed SW/1 -> Input Output Mech E&P Nm radps/2, radps2rpm/1, clutch engage + disengage_torque/4(current_spd_radps), Mech E&P Nm radps/2, eps/1, Bus Creator/6, spd_in_radps/1  "tc_spd_in_radps"
  K factor [RPM / sqrt(Nm)]/1 -> to datalog with base name2/1, Product/1
  Product7/1 -> torque ratio/1, to datalog with base name/1, K factor [RPM / sqrt(Nm)]/1, pos = driving neg = coasting/1
  " torque converter engine load SW"/1 -> Input Output Mech E&P Nm radps/1
  Sum1/1 -> " torque converter engine load SW"/3
  Product6/1 -> " torque converter input speed integrator  (integrate when slipping)"/1
  TC Initial Speed/1 -> " torque converter input speed integrator  (integrate when slipping)"/3
  iner_in_kgm2/1 -> Sum6/1
  Bus Selector/1 -> Saturation/1  "<tcc_lockup_cmd_bool>"
  Sum6/1 -> clutch engage + disengage_torque/5(iner_in_kgm2), Product6/2, torque converter inertia SW/2
  clutch engage + disengage_torque/1(tcc_torque_Nm) -> Sum2/1, Sum5/1  "tcc_torque"
  Sum2/1 -> torque converter trque SW/3
  Product2/1 -> Sum2/2  "hydrodynamic_output_torque"
  Delayed Lockup/1(Lockup) -> " torque converter engine load SW"/2, " torque converter input speed integrator  (integrate when slipping)"/2, torque converter  speed SW/2, torque converter inertia SW/1, torque converter trque SW/2, Bus Creator/2  "tcc_lockup_bool"
  eps/1 -> Product7/2  "impeller_speed"
  pos/1 -> Product7/1  "turbine_speed"
  Bus Creator/1 -> bus_out/1  "torque_converter"
  Sum5/1 -> Sum1/1, Sum3/2, Bus Creator/3  "unlocked_load_Nm"
  Rate Limiter/1 -> Bus Creator/1, Delayed Lockup/1(Engage), to datalog with base name3/1, clutch engage + disengage_torque/1(engage)  "tcc_engage_norm"
  trans_bus/1 -> Bus Selector/1, dynamic lookup/1
  spd_out_radps/1 -> radps2rpm1/1, Input Output Mech E&P Nm radps/5, Bus Creator/7, pos/1, clutch engage + disengage_torque/3(final_spd_radps), torque converter  speed SW/1, TC Initial Speed/1  "tc_spd_out_radps"
  trq_in_Nm/1 -> Subtract2/1, Bus Creator/4, " torque converter engine load SW"/1  "tc_trq_in_Nm"
  Constant/1 -> efficiency multiplier/1
  efficiency multiplier/1 -> torque converter trque SW/1

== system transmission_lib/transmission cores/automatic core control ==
  system_bus : Inport
  Bus Creator : BusCreator  Inputs=2
  Bus Selector : BusSelector  OutputSignals=signal1.control.gear_num,signal1.trans.trans_core.gearbox.gb_curr_gear
  Compare To Zero : simulink/Logic and Bit Operations/Compare To Zero  relop=>  OutDataTypeStr=boolean  ZeroCross=off
  Relational Operator : RelationalOperator  Operator=>  OutDataTypeStr=boolean
  to datalog1 : general_lib/to datalog  VarName=transmission__selected_gear_num  WorkspaceName=datalog__transmission__selected_gear_num  VerboseLevel=1  VerboseSignal=REVS.verbose
  bus_out : Outport
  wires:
  Compare To Zero/1 -> Bus Creator/1  "driveline_engaged_bool"
  Bus Creator/1 -> bus_out/1  "ctrl"
  system_bus/1 -> Bus Selector/1
  Bus Selector/1 -> Compare To Zero/1, Relational Operator/1, to datalog1/1  "<gear_num>"
  Bus Selector/2 -> Relational Operator/2  "<gb_curr_gear>"
  Relational Operator/1 -> Bus Creator/2  "eng_comp_iner_enable"

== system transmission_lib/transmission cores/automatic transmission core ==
  trans_bus : Inport
  trq_in_Nm : Inport  Port=2
  iner_in_kgm2 : Inport  Port=3
  spd_out_radps : Inport  Port=4
  Bus Creator : BusCreator  Inputs=3
  gearbox : transmission_lib/transmission components/gearbox  GearboxBaseName=gearbox  gear=transmission.gear  OutputSignals=gear_num
  bus_out : Outport
  trq_out_Nm : Outport  Port=2
  iner_out_kgm2 : Outport  Port=3
  spd_in_radps : Outport  Port=4
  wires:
  trq_in_Nm/1 -> gearbox/2
  iner_in_kgm2/1 -> gearbox/3
  spd_out_radps/1 -> Bus Creator/3, gearbox/4  "trans_spd_out_radps"
  Bus Creator/1 -> bus_out/1  "trans"
  trans_bus/1 -> gearbox/1
  gearbox/4 -> Bus Creator/2, spd_in_radps/1  "trans_spd_in_radps"
  gearbox/3 -> iner_out_kgm2/1
  gearbox/2 -> trq_out_Nm/1
  gearbox/1 -> Bus Creator/1  "gearbox"

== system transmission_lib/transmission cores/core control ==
  note: 1) Only subsystems can be added as variant choices at this level 2) Blocks cannot be connected at this level as connectivity is automatically determined at simulation, based on the active variant
  system_bus : Inport
  automatic core control : transmission_lib/transmission cores/automatic core control  VariantControl=(transmission_type == enum_transmission_type.automatic)
  dct core control : transmission_lib/transmission cores/dct core control  VariantControl=(transmission_type == enum_transmission_type.DCT)
  bus_out : Outport
